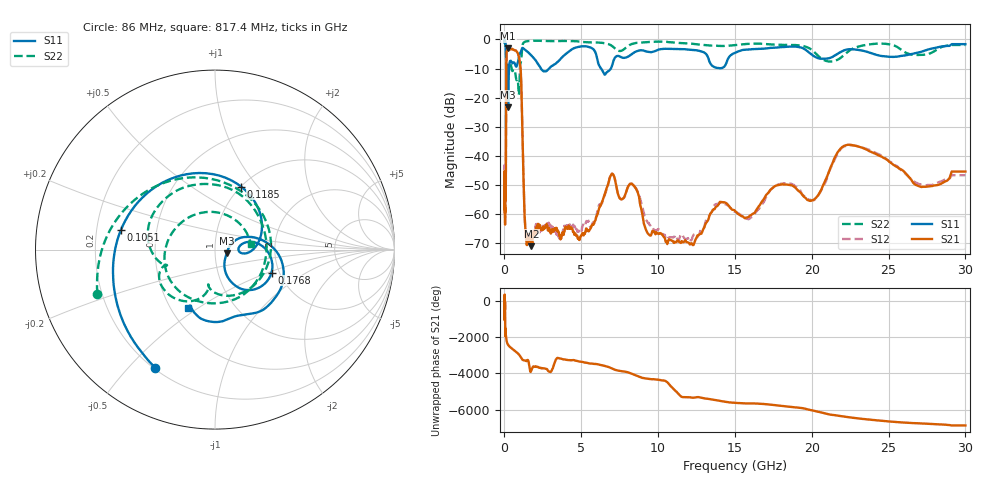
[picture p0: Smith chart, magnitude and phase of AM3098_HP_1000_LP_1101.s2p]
! Date/Time: Thu, Feb 28, 2019 8:40 AM
! Network Analyzer: Agilent Technologies E8364B Rev: A.07.50.67
! Sweep from 0.010 to 30.000 GHz, 1601 Points, Sweep Type: LOG
! Power Supply: 5.023 V, 0.002 A
# Hz S DB R 50
!freq MagS11 AngS11 MagS21 AngS21 MagS12 AngS12 MagS22 AngS22
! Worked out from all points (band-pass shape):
!   1601 points, 10 MHz to 30 GHz, reference 50 ohm
!   highest |S21| = -3.10 dB at 241.1 MHz (marker M1); lowest = -70.9 dB at 1.758 GHz (marker M2)
!   |S21| within 3 dB of the highest: 127.9 MHz to 943.2 MHz (815.3 MHz wide, 152 % of centre)
!   lowest |S11| = -23.4 dB at 238.7 MHz (marker M3), VSWR 1.15, Z = 56.8 - j2.41 ohm
!   |S11| at or under -10 dB: 192 MHz to 298.9 MHz (106.9 MHz wide, 43.5 % of centre); 2.371 GHz to 2.905 GHz (533.5 MHz wide, 20.2 % of centre); 6.286 GHz to 6.926 GHz (639.8 MHz wide, 9.69 % of centre)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
!   |S22| runs from -19.0 to -0.4 dB; largest |S21 - S12| = 0.011
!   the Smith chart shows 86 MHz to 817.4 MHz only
!   S11 on the Smith chart (normalised r, x): 86 MHz: 0.21, -0.60; 105.1 MHz: 0.31, +0.09; 118.5 MHz: 1.00, +0.82; 176.8 MHz: 1.82, -0.53; 817.4 MHz: 0.61, -0.46
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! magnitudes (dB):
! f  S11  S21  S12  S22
! 10 MHz  -0.4  -46.1  -44.4  -0.6
! 38.04 MHz  -0.5  -57.6  -58.2  -1.0
! 86 MHz  -2.6  -51.6  -54.0  -3.1
! 105.1 MHz  -5.4  -27.2  -27.3  -7.0
! 118.5 MHz  -8.4  -10.8  -10.8  -10.3
! 144.7 MHz  -16.9  -4.3  -4.2  -13.2
! 176.8 MHz  -9.4  -3.7  -3.7  -8.9
! 238.7 MHz  -23.4  -3.1  -3.1  -11.0
! 241.1 MHz  -23.2  -3.1  -3.0  -10.9
! 317.5 MHz  -8.7  -3.3  -3.3  -8.3
! 550.5 MHz  -8.1  -3.5  -3.4  -10.7
! 817.4 MHz  -8.9  -4.3  -4.2  -13.9
! 1.066 GHz  -4.3  -11.4  -11.4  -7.9
! 1.382 GHz  -3.7  -66.9  -67.2  -0.7
! 1.758 GHz  -5.6  -70.9  -66.6  -0.5
! 2.084 GHz  -7.6  -64.7  -63.9  -0.5
! 4.952 GHz  -2.4  -67.6  -66.3  -0.8
! 7.926 GHz  -6.2  -52.3  -52.8  -2.7
! 11.89 GHz  -3.5  -69.6  -68.4  -1.4
! 20.1 GHz  -5.6  -55.1  -55.3  -4.0
! 22.56 GHz  -3.4  -36.2  -36.4  -3.5
! 30 GHz  -1.6  -45.3  -46.6  -1.9
